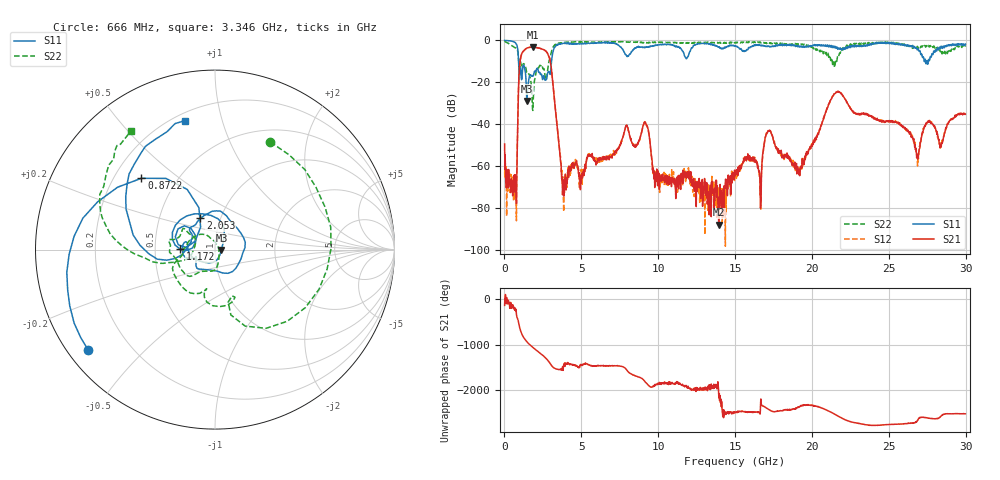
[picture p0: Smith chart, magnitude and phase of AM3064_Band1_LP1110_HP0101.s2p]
# Hz S DB R 50.0
!freq dBS11 angS11 dBS21 angS21 dBS12 angS12 dBS22 angS22
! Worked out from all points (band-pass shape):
!   1600 points, 10 MHz to 29.98 GHz, reference 50 ohm
!   highest |S21| = -3.19 dB at 1.828 GHz (marker M1); lowest = -87.9 dB at 13.94 GHz (marker M2)
!   |S21| within 3 dB of the highest: 1.134 GHz to 2.804 GHz (1.67 GHz wide, 84.8 % of centre)
!   lowest |S11| = -28.9 dB at 1.453 GHz (marker M3), VSWR 1.07, Z = 53.7 - j0.151 ohm
!   |S11| at or under -10 dB: 917.1 MHz to 3.062 GHz (2.145 GHz wide, 108 % of centre); 27.39345 GHz to 27.45917 GHz (65.72 MHz wide, 0.24 % of centre); 27.48785 GHz to 27.56297 GHz (75.12 MHz wide, 0.273 % of centre)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
!   |S22| runs from -33.4 to -0.3 dB; largest |S21 - S12| = 0.011
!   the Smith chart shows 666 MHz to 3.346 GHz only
!   S11 on the Smith chart (normalised r, x): 666 MHz: 0.06, -0.34; 872.2 MHz: 0.31, +0.37; 1.172 GHz: 0.68, +0.00; 2.053 GHz: 0.80, +0.29; 3.346 GHz: 0.24, +0.76
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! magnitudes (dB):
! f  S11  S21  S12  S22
! 10 MHz  0.0  -49.4  -62.9  -0.3
! 666 MHz  -0.9  -72.3  -68.5  -3.4
! 872.2 MHz  -4.9  -36.3  -36.4  -5.6
! 1.172 GHz  -14.3  -5.7  -5.6  -12.4
! 1.453 GHz  -28.9  -3.7  -3.6  -15.2
! 1.828 GHz  -16.9  -3.2  -3.2  -32.9
! 2.053 GHz  -14.3  -3.4  -3.4  -15.0
! 2.897 GHz  -14.8  -7.7  -7.7  -10.0
! 3.346 GHz  -2.6  -35.3  -35.2  -1.8
! 3.852 GHz  -1.4  -68.4  -81.7  -1.1
! 5.015 GHz  -1.4  -65.6  -68.0  -0.6
! 9.157 GHz  -3.3  -39.2  -38.9  -1.1
! 10 GHz  -2.2  -62.4  -64.6  -0.9
! 13.94 GHz  -3.1  -87.9  -76.8  -1.1
! 15 GHz  -2.7  -64.6  -63.3  -1.3
! 16.62 GHz  -2.1  -66.7  -65.1  -0.9
! 17.18 GHz  -2.7  -43.3  -43.2  -1.3
! 19.99 GHz  -2.9  -49.7  -50.1  -3.1
! 21.64 GHz  -3.4  -24.6  -24.7  -8.6
! 25 GHz  -1.0  -38.6  -38.3  -1.2
! 26.87 GHz  -4.4  -56.6  -59.8  -2.9
! 29.98 GHz  -1.8  -35.2  -35.0  -3.0
